FUNCTION_BLOCK FB85
TITLE =Set Velocity Profile
//*****************************************************************************
//* maxon motor ag
//* R&D
//* all rights reserved
//*****************************************************************************
//* Summary:  Set velocity profile
//*
//* Remarks:
//*
//* Created under: STEP7 REV5.2+SP1
//*****************************************************************************
//* History:
//* 19.05.2004 | INA   first release
//*
//*
//*****************************************************************************
//

AUTHOR:INA
FAMILY:ProVeloM
NAME:SetVeloP
VERSION:00.01


VAR_INPUT

Write : BOOL //A rising edge start the command

  NodeID : BYTE //Adress of the maxon device

  ProfileAcceleration : DWORD //Velocity Profile Acceleration

  ProfileDeceleration : DWORD //Velocity Profile Deceleration

END_VAR
VAR_OUTPUT
  Done : BOOL //Data valid flag is TRUE if data were available

  Err : BOOL //Error flag is TRUE if an Error has occured, see ErrNo for more details

  ErrNo : DINT //Contains detailed error information

END_VAR
VAR
  xEdgeMerker : BOOL //Edge Merker

  xEdgeFlag : BOOL //Edge Flag

  xStep : INT
END_VAR

BEGIN

NETWORK
TITLE = Activate the service function
//

// SDO Write "Set Velocity Profile"

       U    #Write
       FP   #xEdgeFlag                   // recognize a positiv edge of the Read signal
       =    #xEdgeMerker                 // and set the xEdgeMerker for one cycle to true

       L    #xStep
       L    0
       ==I
       U    #xEdgeMerker
       SPB  nstp                         // iStep = 1 -> fnc1

       L    #xStep                       // jump list
       SPL  List
       SPA  rdef
       SPA  fnc1
       SPA  fncE
List  :SPA  rdef

rdef  :NOP  0
       R    #Done                        // reset Done
       R    #Err
       L    0
       T    #xStep                       // iStep = 0
       SPA  end

fnc1  :NOP  0
       CALL FC16
         NodeID:=#NodeID
         Index:=DW#16#00006083
         SubIndex:=DW#16#00000000
         ValueIn:=#ProfileAcceleration
         RET_VAL:=#Done
         Err:=#Err
         ErrNo:=#ErrNo

       L    1
       U    #Err
       SPB  fncE

       NOP  0
       CALL FC16
         NodeID:=#NodeID
         Index:=DW#16#00006084
         SubIndex:=DW#16#00000000
         ValueIn:=#ProfileDeceleration
         RET_VAL:=#Done
         Err:=#Err
         ErrNo:=#ErrNo

       L    1
       U    #Err
       SPB  fncE

       SPA  nstp                         // iStep = 2 -> fncE

fncE  :NOP  0
       L    0
       T    #xStep
       SPA  end

nstp  :NOP  0
       L    #xStep
       INC            1
       T    #xStep

end   :NOP  0
END_FUNCTION_BLOCK
